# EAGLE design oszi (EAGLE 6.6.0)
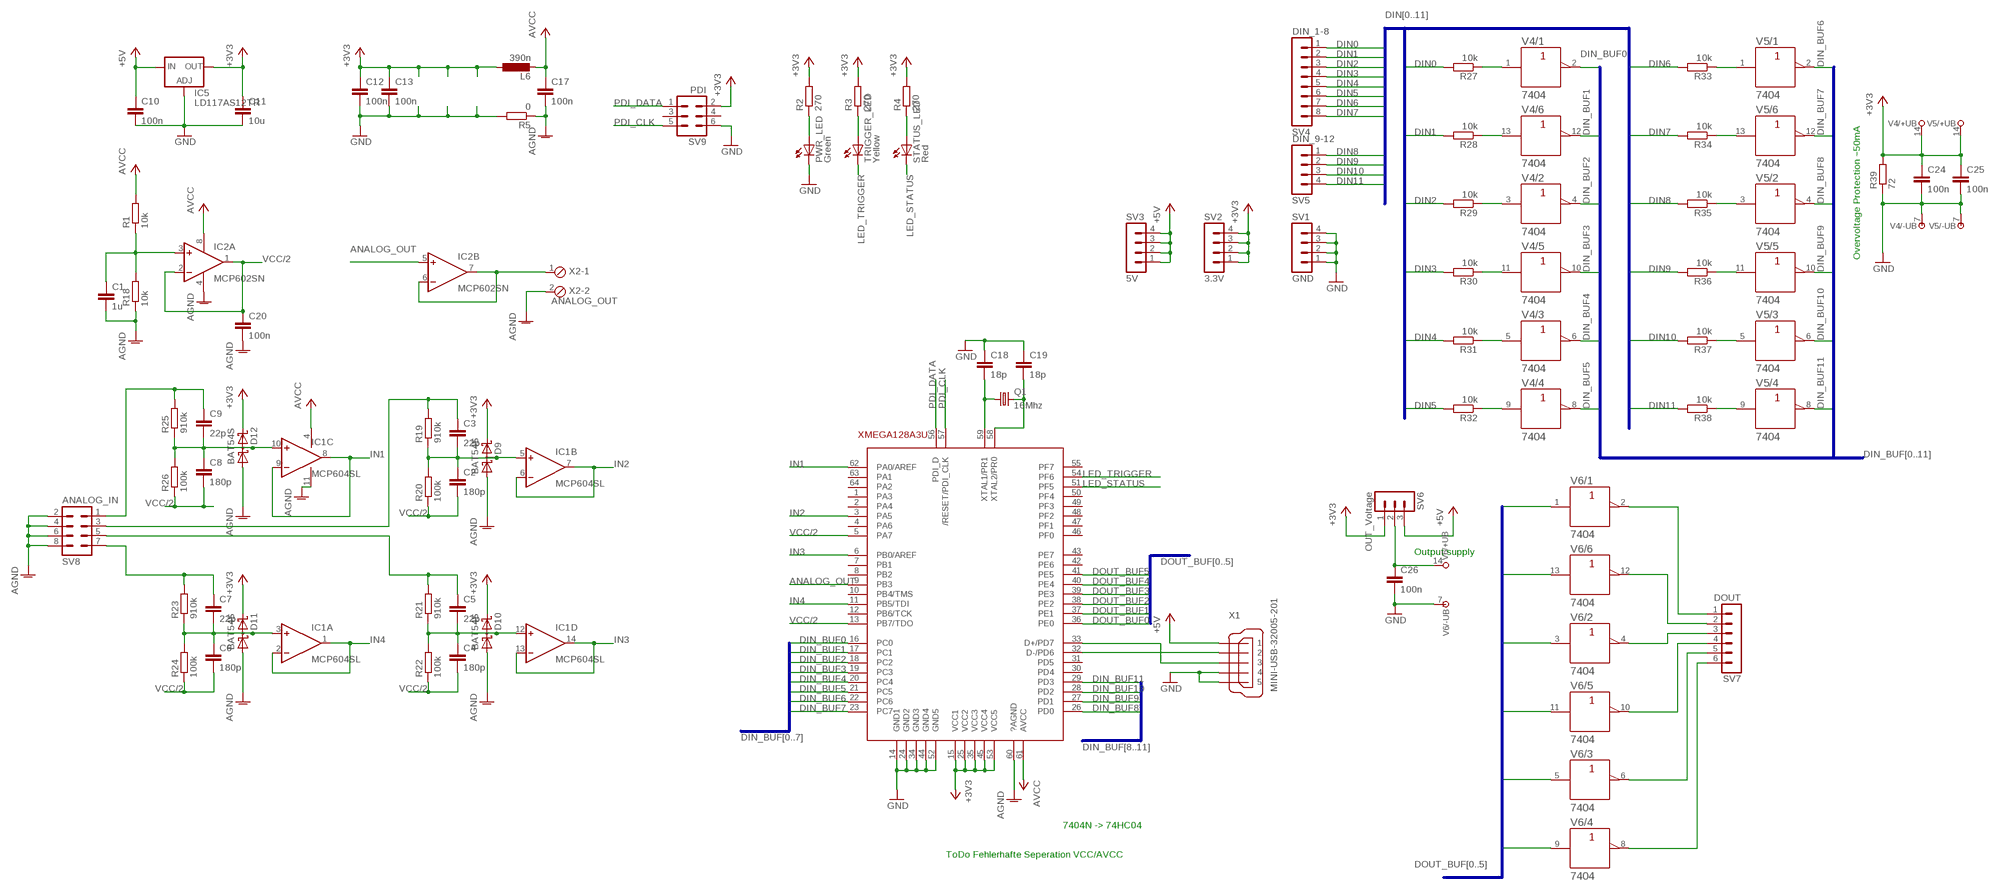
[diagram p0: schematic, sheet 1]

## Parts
C1  1u  C-EUC0805  [C0805]
C2  180p  C-EUC0805  [C0805]
C3  22p  C-EUC0805  [C0805]
C4  180p  C-EUC0805  [C0805]
C5  22p  C-EUC0805  [C0805]
C6  180p  C-EUC0805  [C0805]
C7  22p  C-EUC0805  [C0805]
C8  180p  C-EUC0805  [C0805]
C9  22p  C-EUC0805  [C0805]
C10  100n  C-EUC0805  [C0805]
C11  10u  C-EUC0805  [C0805]
C12  100n  C-EUC0805  [C0805]
C13  100n  C-EUC0805  [C0805]
C17  100n  C-EUC0805  [C0805]
C18  18p  C-EUC0805  [C0805]
C19  18p  C-EUC0805  [C0805]
C20  100n  C-EUC0805  [C0805]
C24  100n  C-EUC0805  [C0805]
C25  100n  C-EUC0805  [C0805]
C26  100n  C-EUC0805  [C0805]
D9  BAT54S  [SOT23]
D10  BAT54S  [SOT23]
D11  BAT54S  [SOT23]
D12  BAT54S  [SOT23]
IC1  MCP604SL  [SO14]
IC2  MCP602SN  [SO08]
IC5  LD117AS12TR  [SOT223]
L6  390n  L-EUL2825P  [L2825P]
PWR_LED  Green  LEDSML0805  [SML0805]
Q1  16Mhz  CRYSTALHC49UP  [HC49UP]
R1  10k  R-EU_R0805  [R0805]
R2  270  R-EU_R0805  [R0805]
R3  270  R-EU_R0805  [R0805]
R4  270  R-EU_R0805  [R0805]
R5  0  R-EU_R0805  [R0805]
R18  10k  R-EU_R0805  [R0805]
R19  910k  R-EU_R0805  [R0805]
R20  100k  R-EU_R0805  [R0805]
R21  910k  R-EU_R0805  [R0805]
R22  100k  R-EU_R0805  [R0805]
R23  910k  R-EU_R0805  [R0805]
R24  100k  R-EU_R0805  [R0805]
R25  910k  R-EU_R0805  [R0805]
R26  100k  R-EU_R0805  [R0805]
R27  10k  R-EU_R0805  [R0805]
R28  10k  R-EU_R0805  [R0805]
R29  10k  R-EU_R0805  [R0805]
R30  10k  R-EU_R0805  [R0805]
R31  10k  R-EU_R0805  [R0805]
R32  10k  R-EU_R0805  [R0805]
R33  10k  R-EU_R0805  [R0805]
R34  10k  R-EU_R0805  [R0805]
R35  10k  R-EU_R0805  [R0805]
R36  10k  R-EU_R0805  [R0805]
R37  10k  R-EU_R0805  [R0805]
R38  10k  R-EU_R0805  [R0805]
R39  72  R-EU_R0805  [R0805]
STATUS_LED  Red  LEDSML0805  [SML0805]
SV1  GND  MA04-1  [MA04-1]
SV2  3.3V  MA04-1  [MA04-1]
SV3  5V  MA04-1  [MA04-1]
SV4  DIN_1-8  MA08-1  [MA08-1]
SV5  DIN_9-12  MA04-1  [MA04-1]
SV6  OUT_Voltage  MA03-1  [MA03-1]
SV7  DOUT  MA06-1  [MA06-1]
SV8  ANALOG_IN  MA04-2  [MA04-2]
SV9  PDI  ML6  [ML6]
TRIGGER_LED  Yellow  LEDSML0805  [SML0805]
U$1  XMEGA128A3U  [TQFP64]
V4  7404  [SO14]
V5  7404  [SO14]
V6  7404  [SO14]
X1  MINI-USB-32005-201  [32005-201]
X2  ANALOG_OUT  MPT2  [2POL254]

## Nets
+3V3: C11.1 C12.1 C13.1 C24.1 C25.1 D9.2(C2) D10.2(C2) D11.2(C2) D12.2(C2) IC5.4(OUT) L6.1 R2.2 R3.2 R4.2 R39.2 SV2.1 SV2.2 SV2.3 SV2.4 SV6.1 SV9.2 U$1.15(VCC1) U$1.25(VCC2) U$1.35(VCC3) U$1.45(VCC4) U$1.53(VCC5) V4.14(/+UB:+UB) V5.14(/+UB:+UB)
+5V: C10.1 IC5.3(IN) SV3.1 SV3.2 SV3.3 SV3.4 SV6.3 X1.1
AGND: C1.2 C17.2 C20.2 D9.1(A1) D10.1(A1) D11.1(A1) D12.1(A1) IC1.11(P:V-) IC2.4(P:V-) R5.1 R18.1 SV8.2 SV8.4 SV8.6 SV8.8 U$1.60(?AGND) X2.2
ANALOG_OUT: IC2.5(B:+IN) U$1.9(PB3)
DIN0: R27.2 SV4.1
DIN1: R28.2 SV4.2
DIN2: R29.2 SV4.3
DIN3: R30.2 SV4.4
DIN4: R31.2 SV4.5
DIN5: R32.2 SV4.6
DIN6: R33.2 SV4.7
DIN7: R34.2 SV4.8
DIN8: R35.2 SV5.1
DIN9: R36.2 SV5.2
DIN10: R37.2 SV5.3
DIN11: R38.2 SV5.4
DIN_BUF0: U$1.16(PC0) V4.2(/1:Y)
DIN_BUF1: U$1.17(PC1) V4.12(/6:Y)
DIN_BUF2: U$1.18(PC2) V4.4(/2:Y)
DIN_BUF3: U$1.19(PC3) V4.10(/5:Y)
DIN_BUF4: U$1.20(PC4) V4.6(/3:Y)
DIN_BUF5: U$1.21(PC5) V4.8(/4:Y)
DIN_BUF6: U$1.22(PC6) V5.2(/1:Y)
DIN_BUF7: U$1.23(PC7) V5.12(/6:Y)
DIN_BUF8: U$1.26(PD0) V5.4(/2:Y)
DIN_BUF9: U$1.27(PD1) V5.10(/5:Y)
DIN_BUF10: U$1.28(PD2) V5.6(/3:Y)
DIN_BUF11: U$1.29(PD3) V5.8(/4:Y)
DOUT_BUF0: U$1.36(PE0) V6.1(/1:A)
DOUT_BUF1: U$1.37(PE1) V6.13(/6:A)
DOUT_BUF2: U$1.38(PE2) V6.3(/2:A)
DOUT_BUF3: U$1.39(PE3) V6.11(/5:A)
DOUT_BUF4: U$1.40(PE4) V6.5(/3:A)
DOUT_BUF5: U$1.41(PE5) V6.9(/4:A)
GND: C10.2 C11.2 C12.2 C13.2 C18.1 C19.1 C24.2 C25.2 C26.2 IC5.1(ADJ) PWR_LED.C R5.2 R39.1 SV1.1 SV1.2 SV1.3 SV1.4 SV9.6 U$1.14(GND1) U$1.24(GND2) U$1.34(GND3) U$1.44(GND4) U$1.52(GND5) V4.7(/-UB:-UB) V5.7(/-UB:-UB) V6.7(/-UB:-UB) X1.4 X1.5
IN1: IC1.8(C:OUT) IC1.9(C:-IN) U$1.62(PA0/AREF)
IN2: IC1.6(B:-IN) IC1.7(B:OUT) U$1.3(PA5)
IN3: IC1.13(D:-IN) IC1.14(D:OUT) U$1.6(PB0/AREF)
IN4: IC1.1(A:OUT) IC1.2(A:-IN) U$1.11(PB5/TDI)
LED_STATUS: STATUS_LED.C U$1.51(PF5)
LED_TRIGGER: TRIGGER_LED.C U$1.54(PF6)
N$1: U$1.32(D-/PD6) X1.2
N$2: U$1.33(D+/PD7) X1.3
N$3: PWR_LED.A R2.1
N$4: C1.1 IC2.3(A:+IN) R1.1 R18.2
N$5: R3.1 TRIGGER_LED.A
N$6: R33.1 V5.1(/1:A)
N$8: R4.1 STATUS_LED.A
N$21: C2.1 C3.2 D9.3(C1A2) IC1.5(B:+IN) R19.1 R20.2
N$24: C4.1 C5.2 D10.3(C1A2) IC1.12(D:+IN) R21.1 R22.2
N$26: C5.1 R21.2 SV8.5
N$27: C6.1 C7.2 D11.3(C1A2) IC1.3(A:+IN) R23.1 R24.2
N$29: C7.1 R23.2 SV8.7
N$30: C8.1 C9.2 D12.3(C1A2) IC1.10(C:+IN) R25.1 R26.2
N$32: C9.1 R25.2 SV8.1
N$33: IC2.6(B:-IN) IC2.7(B:OUT) X2.1
N$34: R27.1 V4.1(/1:A)
N$35: R28.1 V4.13(/6:A)
N$36: R29.1 V4.3(/2:A)
N$37: R30.1 V4.11(/5:A)
N$38: R31.1 V4.5(/3:A)
N$39: R32.1 V4.9(/4:A)
N$41: R34.1 V5.13(/6:A)
N$42: R35.1 V5.3(/2:A)
N$43: R36.1 V5.11(/5:A)
N$44: R37.1 V5.5(/3:A)
N$45: R38.1 V5.9(/4:A)
N$46: C18.2 Q1.1 U$1.59(XTAL1/PR1)
N$47: C26.1 SV6.2 V6.14(/+UB:+UB)
N$48: SV7.1 V6.2(/1:Y)
N$49: SV7.2 V6.12(/6:Y)
N$50: SV7.3 V6.4(/2:Y)
N$51: SV7.4 V6.10(/5:Y)
N$52: SV7.5 V6.6(/3:Y)
N$53: SV7.6 V6.8(/4:Y)
N$54: C3.1 R19.2 SV8.3
N$55: C19.2 Q1.2 U$1.58(XTAL2/PR0)
PDI_CLK: SV9.5 U$1.57(/RESET/PDI_CLK)
PDI_DATA: SV9.1 U$1.56(PDI_D)
VCC: C17.1 IC1.4(P:V+) IC2.8(P:V+) L6.2 R1.2 U$1.61(AVCC) ; supply symbol labelled AVCC
VCC/2: C2.2 C4.2 C6.2 C8.2 C20.1 IC2.1(A:OUT) IC2.2(A:-IN) R20.1 R22.1 R24.1 R26.1 U$1.5(PA7) U$1.13(PB7/TDO)
Unconnected: SV9.3 SV9.4 U$1.1(PA3) U$1.2(PA4) U$1.4(PA6) U$1.7(PB1) U$1.8(PB2) U$1.10(PB4/TMS) U$1.12(PB6/TCK) U$1.30(PD4) U$1.31(PD5) U$1.42(PE6) U$1.43(PE7) U$1.46(PF0) U$1.47(PF1) U$1.48(PF2) U$1.49(PF3) U$1.50(PF4) U$1.55(PF7) U$1.63(PA1) U$1.64(PA2)

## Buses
DIN[0..11]
DIN_BUF[0..11]
DOUT_BUF[0..5]
DIN_BUF[0..7]
DIN_BUF[8..11]

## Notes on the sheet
- Overvoltage Protection ~50mA
- Output supply
- 7404N -> 74HC04
- ToDo Fehlerhafte Seperation VCC/AVCC

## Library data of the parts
C1-C13 C17-C20 C24-C26 = resistor:C-EU: CAPACITOR, European symbol
D9-D12 = diode:BAT54S: Schottky Diodes Pin connection corrected 2011-05-04 Source: Fairchild .. BAT54.pdf
IC1 = linear:MCP604: Quad Op Amp 2.7V to 6.0V Single Supply CMOS Source: http://ww1.microchip.com/downloads/en/DeviceDoc/21314g.pdf
IC2 = linear:MCP602: Single Op Amp 2.7V to 6.0V Single Supply CMOS Source: http://ww1.microchip.com/downloads/en/DeviceDoc/21314g.pdf
IC5 = v-reg:LD117A?*: Low drop fixed and adjustable positive voltage regulators 1 A Source: http://www.st.com/stonline/products/literature/ds/7194/ld1117axx.pdf
L6 = resistor:L-EU: INDUCTOR, European symbol
PWR_LED STATUS_LED TRIGGER_LED = led:LED: LED
Q1 = crystal:CRYSTAL: CRYSTAL; OC_FARNELL: unknown; OC_NEWARK: unknown
R1-R5 R18-R39 = resistor:R-EU_: RESISTOR, European symbol
SV1-SV3 SV5 = con-lstb:MA04-1: PIN HEADER; OC_FARNELL: unknown; OC_NEWARK: unknown
SV4 = con-lstb:MA08-1: PIN HEADER; OC_FARNELL: unknown; OC_NEWARK: unknown
SV6 = con-lstb:MA03-1: PIN HEADER; OC_FARNELL: unknown; OC_NEWARK: unknown
SV7 = con-lstb:MA06-1: PIN HEADER; OC_FARNELL: unknown; OC_NEWARK: unknown
SV8 = con-lstb:MA04-2: PIN HEADER; OC_FARNELL: unknown; OC_NEWARK: unknown
SV9 = con-ml:ML6: HARTING; OC_FARNELL: unknown; OC_NEWARK: unknown
U$1 = Wasle:XMEGA128A3U
V4-V6 = Wasle:74*04: Hex INVERTER
X1 = con-cypressindustries:MINI-USB-: MINI USB-B Conector Source: www.cypressindustries.com; OC_FARNELL: unknown; OC_NEWARK: unknown
X2 = con-phoenix-254:MPT2: PHOENIX CONNECTOR; OC_FARNELL: unknown; OC_NEWARK: unknown

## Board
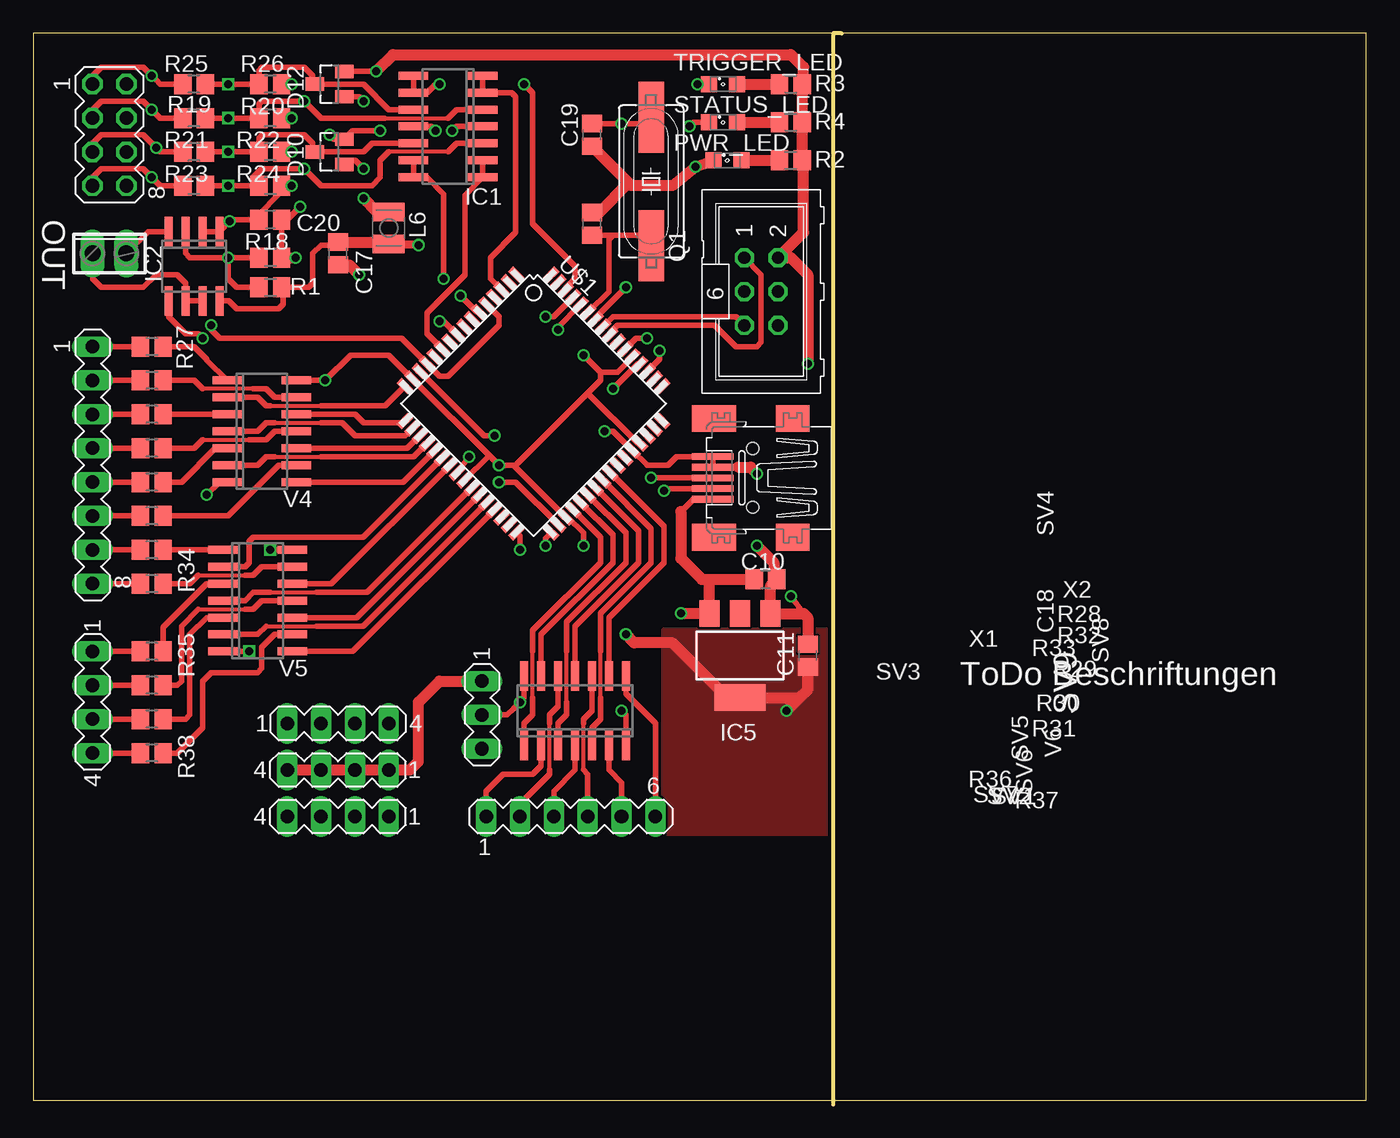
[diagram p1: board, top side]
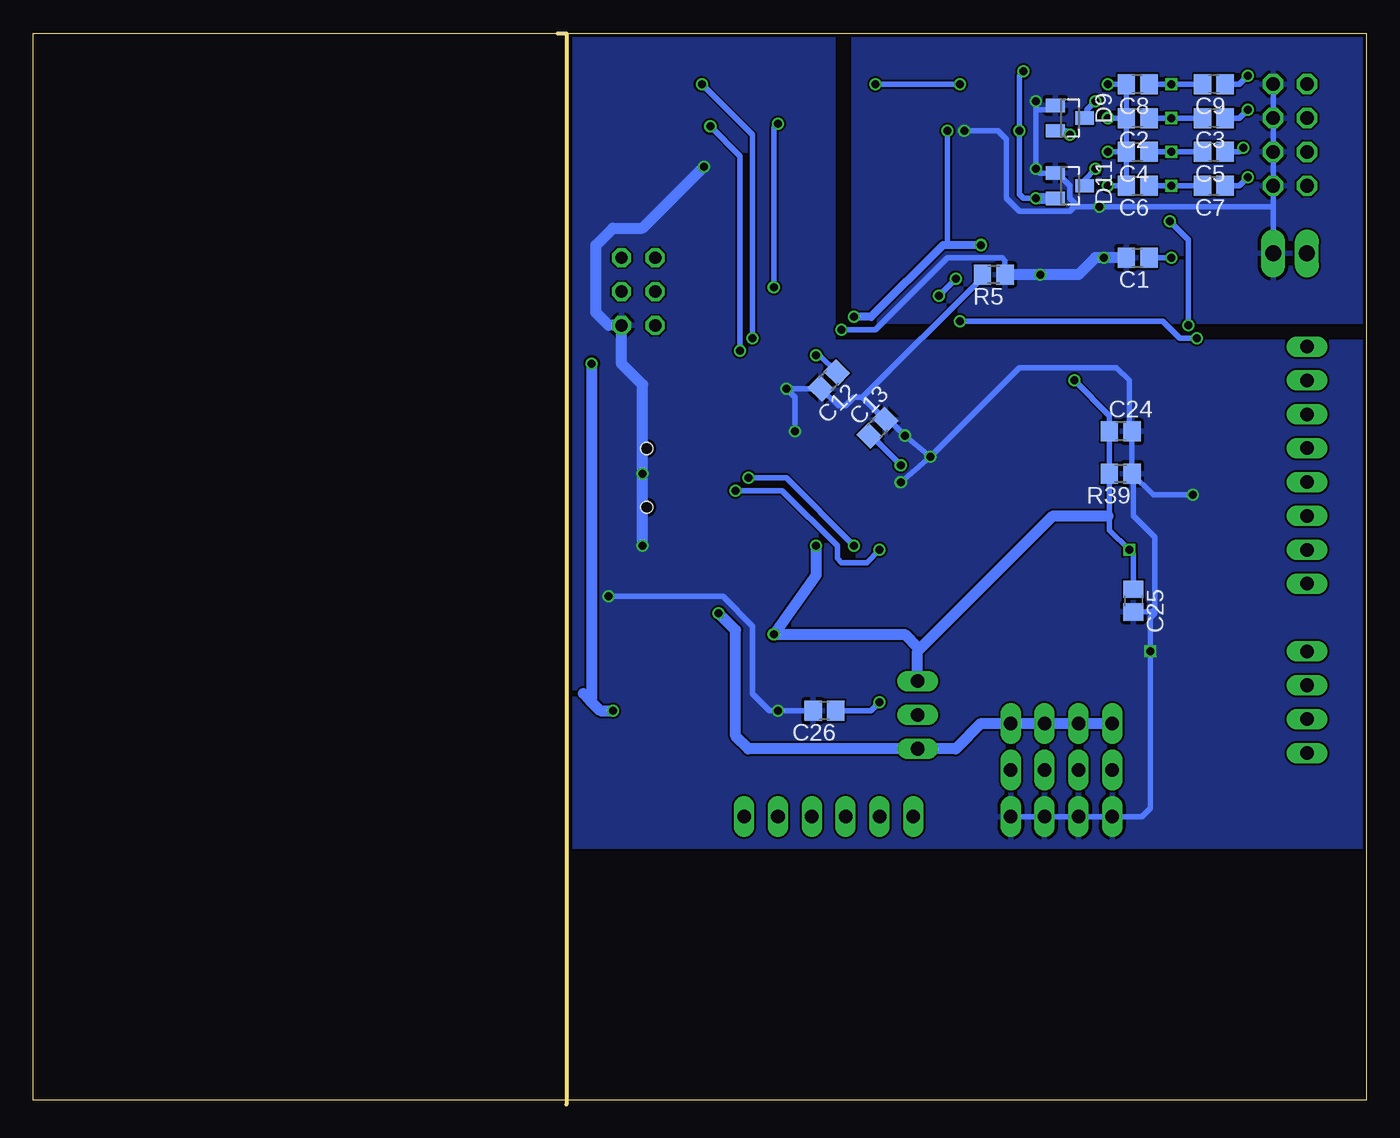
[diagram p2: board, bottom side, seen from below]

Size 100 x 80.33 mm. Coordinates in mm from the lower left corner, seen from the top.
Outline: 60.64,80.33 60.01,80.33 60.01,0
Outline: 0,0.32 100,0.32 100,80.32 0,80.32 0,0.32
Copper layers (1*16): Top 0.035mm / dielectric 1.5mm / Bottom 0.035mm
Design rules "Elecrow_2-layer_eagle_rule": minimum track width 6mil, minimum drill 12mil, track to track 6mil, track to pad 6mil, pad to pad 6mil, via to via 6mil, smd to smd 0mil, copper to edge 10mil, drill to drill 10mil, minimum pad ring 10mil, minimum via ring 6mil, stop-mask expansion 2mil, vias tented up to drill 100mil, thermal gap 10mil

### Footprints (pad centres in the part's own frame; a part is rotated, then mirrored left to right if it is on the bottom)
C0805 = smd 1.3 x 1.5: 1 -0.85,0; 2 0.85,0
SOT23 = smd 1 x 1.4: 1 -0.95,-1.1; 2 0.95,-1.1; 3 0,1.1
SO14 = smd 0.6 x 2.2: 1 -3.81,-2.6; 2 -2.54,-2.6; 3 -1.27,-2.6; 4 0,-2.6; 5 1.27,-2.6; 6 2.54,-2.6; 7 3.81,-2.6; 8 3.81,2.6; 9 2.54,2.6; 10 1.27,2.6; 11 0,2.6; 12 -1.27,2.6; 13 -2.54,2.6; 14 -3.81,2.6
SO08 = smd 0.6 x 2.2: 1 -1.905,-2.6; 2 -0.635,-2.6; 3 0.635,-2.6; 4 1.905,-2.6; 5 1.905,2.6; 6 0.635,2.6; 7 -0.635,2.6; 8 -1.905,2.6
SOT223 = smd 1.5 x 2: 1 -2.3,-3.15; 2 0,-3.15; 3 2.3,-3.15 | smd 3.8 x 2: 4 0,3.15
L2825P = smd 1.4 x 2.4: 1 -1.2,0; 2 1.2,0
SML0805 = smd 1.2 x 1.2: A 1.05,0; C -1.05,0
HC49UP = smd 5.334 x 1.93: 1 -4.826,0; 2 4.826,0
R0805 = smd 1.3 x 1.5: 1 -0.85,0; 2 0.85,0
MA04-1 = drill 1.016 long: 1 -3.81,0; 2 -1.27,0; 3 1.27,0; 4 3.81,0
MA08-1 = drill 1.016 long: 1 -8.89,0; 2 -6.35,0; 3 -3.81,0; 4 -1.27,0; 5 1.27,0; 6 3.81,0; 7 6.35,0; 8 8.89,0
MA03-1 = drill 1.016 long: 1 -2.54,0; 2 0,0; 3 2.54,0
MA06-1 = drill 1.016 long: 1 -6.35,0; 2 -3.81,0; 3 -1.27,0; 4 1.27,0; 5 3.81,0; 6 6.35,0
MA04-2 = drill 1.016 octagon: 1 -3.81,-1.27; 2 -3.81,1.27; 3 -1.27,-1.27; 4 -1.27,1.27; 5 1.27,-1.27; 6 1.27,1.27; 7 3.81,-1.27; 8 3.81,1.27
ML6 = drill 0.914 octagon: 1 -2.54,-1.27; 2 -2.54,1.27; 3 0,-1.27; 4 0,1.27; 5 2.54,-1.27; 6 2.54,1.27
TQFP64 = smd 1.194 x 0.559: 1 -7.76,5.905; 2 -7.76,5.118; 3 -7.76,4.331; 4 -7.76,3.543; 5 -7.76,2.756; 6 -7.76,1.968; 7 -7.76,1.181; 8 -7.76,0.394; 9 -7.76,-0.394; 10 -7.76,-1.181; 11 -7.76,-1.968; 12 -7.76,-2.756; 13 -7.76,-3.543; 14 -7.76,-4.331; 15 -7.76,-5.118; 16 -7.76,-5.905; 33 7.76,-5.905; 34 7.76,-5.118; 35 7.76,-4.331; 36 7.76,-3.543; 37 7.76,-2.756; 38 7.76,-1.968; 39 7.76,-1.181; 40 7.76,-0.394; 41 7.76,0.394; 42 7.76,1.181; 43 7.76,1.968; 44 7.76,2.756; 45 7.76,3.543; 46 7.76,4.331; 47 7.76,5.118; 48 7.76,5.905 | smd 0.559 x 1.194: 17 -5.905,-7.76; 18 -5.118,-7.76; 19 -4.331,-7.76; 20 -3.543,-7.76; 21 -2.756,-7.76; 22 -1.968,-7.76; 23 -1.181,-7.76; 24 -0.394,-7.76; 25 0.394,-7.76; 26 1.181,-7.76; 27 1.968,-7.76; 28 2.756,-7.76; 29 3.543,-7.76; 30 4.331,-7.76; 31 5.118,-7.76; 32 5.905,-7.76; 49 5.905,7.76; 50 5.118,7.76; 51 4.331,7.76; 52 3.543,7.76; 53 2.756,7.76; 54 1.968,7.76; 55 1.181,7.76; 56 0.394,7.76; 57 -0.394,7.76; 58 -1.181,7.76; 59 -1.968,7.76; 60 -2.756,7.76; 61 -3.543,7.76; 62 -4.331,7.76; 63 -5.118,7.76; 64 -5.905,7.76
32005-201 = smd 3.1 x 0.5: 1 3,1.6; 2 3,0.8; 3 3,0; 4 3,-0.8; 5 3,-1.6 | smd 2.5 x 2: M1 -3,-4.45; M2 -3,4.45 | smd 3.3 x 2: M3 2.9,4.45; M4 2.9,-4.45 | hole 0.9: 0,2.2; 0,-2.2
2POL254 = drill 1.2 long: 1 -1.27,0; 2 1.27,0

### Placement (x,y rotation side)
C1  17.14,63.5 180 bottom
C2  17.14,73.98 180 bottom
C3  11.43,73.98 180 bottom
C4  17.14,71.44 180 bottom
C5  11.43,71.44 180 bottom
C6  17.14,68.9 180 bottom
C7  11.43,68.9 180 bottom
C8  17.14,76.52 180 bottom
C9  11.43,76.52 180 bottom
C10  54.93,39.37 0 top
C11  58.1,33.66 90 top
C12  40.31,54.29 225 bottom
C13  36.67,50.74 45 bottom
C17  22.86,63.82 270 top
C18  41.91,66.04 270 top
C19  41.91,72.71 90 top
C20  17.78,66.36 0 top
C24  18.41,50.48 0 bottom
C25  17.46,37.78 270 bottom
C26  40.64,29.53 180 bottom
D9  22.23,73.98 270 bottom
D10  22.23,71.44 90 top
D11  22.23,68.9 270 bottom
D12  22.23,76.52 90 top
IC1  31.11,73.34 90 top
IC2  12.06,62.87 180 top
IC5  53.02,33.66 180 top
L6  26.67,65.72 270 top
PWR_LED  52.07,70.8 0 top
Q1  46.35,69.21 90 top
R1  17.78,61.28 0 top
R2  56.83,70.8 0 top
R3  56.83,76.52 0 top
R4  56.83,73.66 0 top
R5  27.94,62.23 180 bottom
R18  17.78,63.5 180 top
R19  12.06,73.98 180 top
R20  17.78,73.98 180 top
R21  12.06,71.44 180 top
R22  17.78,71.44 180 top
R23  12.06,68.9 180 top
R24  17.78,68.9 180 top
R25  12.06,76.52 180 top
R26  17.78,76.52 180 top
R27  8.89,56.83 180 top
R28  8.89,54.29 180 top
R29  8.89,51.75 180 top
R30  8.89,49.21 180 top
R31  8.89,46.67 180 top
R32  8.89,44.13 180 top
R33  8.89,41.59 180 top
R34  8.89,39.05 180 top
R35  8.89,33.97 180 top
R36  8.89,31.43 180 top
R37  8.89,28.89 180 top
R38  8.89,26.35 180 top
R39  18.41,47.31 180 bottom
STATUS_LED  51.75,73.66 0 top
SV1  22.86,21.59 180 top
SV2  22.86,25.08 180 top
SV3  22.86,28.57 0 top
SV4  4.45,47.94 270 top
SV5  4.45,30.16 270 top
SV6  33.66,29.21 270 top
SV7  40.32,21.59 0 top
SV8  5.71,72.71 270 top
SV9  54.61,60.96 270 top
TRIGGER_LED  51.75,76.52 0 top
U$1  37.54,52.56 315 top
V4  17.14,50.48 270 top
V5  16.83,37.78 270 top
V6  40.64,29.53 0 top
X1  53.98,46.99 180 top
X2  5.71,63.82 0 top

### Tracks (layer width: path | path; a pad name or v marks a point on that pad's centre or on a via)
+3V3  (via drill 0.6)
  Top 0.406: v26.04,73.02 23.96,73.02 D10.2 22.54,72.39 v22.23,72.71 | D12.2 v25.72,77.47 | 34.29,48.58 U$1.15 26.66,56.2 23.81,56.2 v21.91,54.29 V4.14 | 34.29,48.58 34.11,48.58 U$1.25 | 34.29,48.58 v34.92,47.94 36.03,47.94 36.11,47.86 | V5.14 v17.78,41.59 | 36.11,47.86 U$1.35 40.12,44.01 41.27,42.86 v41.27,41.91 | U$1.53 44.97,56.08 43.81,54.93 42.55,54.93 | v41.27,56.2 42.55,54.93 | 42.55,54.93 42.55,54.29 41.59,53.34 | 41.59,53.34 36.11,47.86 | U$1.45 45.35,49.58 41.59,53.34 | R3.2 57.78,76.52
  Top 0.813: SV2.4 SV2.3 SV2.2 SV2.1 28.26,25.08 28.89,25.72 28.89,30.16 30.48,31.75 SV6.1 | 57.49,30.51 IC5.4 53.02,30.48 52.07,30.48 47.94,34.61 45.09,34.61 v44.45,35.24 | 57.49,30.51 58.1,31.11 C11.1 | R3.2 R4.2 R2.2 57.78,71.02 57.78,65.41 SV9.2 56.83,63.5 58.1,62.23 v58.1,55.56 | v25.72,77.47 26.99,78.74 56.83,78.74 57.78,77.79 57.78,76.52 | v56.52,29.53 57.49,30.51 | L6.1 25.79,66.93 v24.77,67.95
  Bottom 0.406: v24.77,67.95 25.72,67.95 26.04,68.26 v26.04,73.02 26.04,77.15 v25.72,77.47 | C25.1 17.46,41.28 v17.78,41.59 19.27,43.08 R39.2 C24.1 19.27,51.65 v21.91,54.29 | v41.27,56.2 41.02,56.2 C12.1 | C13.1 37.13,50.14 v34.92,47.94 | D9.2 22.55,73.03 v22.23,72.71
  Bottom 0.813: 33.66,33.97 33.66,34.29 34.61,35.24 v44.45,35.24 41.27,39.69 v41.27,41.91 | 58.74,30.8 58.26,30.32 | 58.26,30.32 57.47,29.53 v56.52,29.53 | v58.1,55.56 58.1,30.48 58.26,30.32 | v24.77,67.95 D11.2 | SV6.1 33.66,33.97 | 33.66,33.97 23.5,44.13 19.37,44.13
  pour Top (no thermals): 47.31,35.56 59.69,35.56 59.69,20.32 47.31,20.32
+5V  (via drill 0.6)
  Top 0.406: X1.1 49.52,45.39 48.58,44.45
  Top 0.813: 48.58,44.45 48.58,40.96 50.16,39.37 50.8,39.37 | 50.8,39.37 C10.1 | 50.8,39.37 50.72,39.29 IC5.3 50.7,36.83 v48.58,36.83
  Bottom 0.813: v48.58,36.83 47.31,35.56 47.31,27.62 46.35,26.67 SV6.3 30.8,26.67 28.89,28.58 SV3.4 SV3.3 SV3.2 SV3.1
AGND  (via drill 0.6)
  Top 0.406: D12.1 24.45,75.57 v24.77,75.25 | v24.77,70.17 24.13,70.8 23.64,70.8 D10.1 | IC2.4 8.63,65.46 X2.2 | R18.1 C20.2 19.05,66.36 v20,67.31 | v39.37,58.1 39.37,58.3 U$1.60 | IC1.11 29.84,73.34 v30.16,73.02
  Top 0.813: C17.2 23.71,62.97 v24.45,62.23 | R18.1 v19.68,63.5
  Bottom 0.406: SV8.2 SV8.4 SV8.6 SV8.8 6.99,67.31 | v24.77,75.25 24.77,74.61 | 24.77,74.61 23.64,74.61 D9.1 | 24.77,74.61 v24.77,70.17 24.45,69.85 D11.1 23.18,69.85 22.23,68.9 22.23,67.94 21.59,67.31 | 6.99,67.31 X2.2 | 6.99,67.31 v20,67.31 21.59,67.31 | 21.59,67.31 21.91,67.31 22.23,66.99 26.04,66.99 26.99,67.94 26.99,72.39 27.62,73.02 v30.16,73.02 | R5.1 27.09,63.29 27.3,63.5 31.43,63.5 36.83,58.1 v39.37,58.1
  Bottom 0.813: R5.1 v24.45,62.23 21.59,62.23 20.32,63.5 v19.68,63.5 C1.2
  pour Bottom: -0.64,81.6 38.42,81.6 38.42,58.74 -0.64,58.74
ANALOG_OUT  (via drill 0.6)
  Top 0.406: IC2.5 10.16,59.05 11.43,57.79 12.38,57.79 v12.7,57.47 | U$1.9 30.8,58.74 v30.48,58.74
  Bottom 0.406: v12.7,57.47 13.97,57.47 15.24,58.74 v30.48,58.74
DIN0
  Top 0.406: R27.2 SV4.1
DIN1
  Top 0.406: R28.2 SV4.2
DIN2
  Top 0.406: SV4.3 R29.2
DIN3
  Top 0.406: SV4.4 R30.2
DIN4
  Top 0.406: SV4.5 R31.2
DIN5
  Top 0.406: SV4.6 R32.2
DIN6
  Top 0.406: SV4.7 R33.2
DIN7
  Top 0.406: SV4.8 R34.2
DIN8
  Top 0.406: SV5.1 R35.2
DIN9
  Top 0.406: SV5.2 R36.2
DIN10
  Top 0.406: SV5.3 R37.2
DIN11
  Top 0.406: SV5.4 R38.2
DIN_BUF0
  Top 0.305: 17.78,52.39 21.59,52.39
  Top 0.406: V4.2 16.83,53.02 17.46,52.39 17.78,52.39 | 21.59,52.39 26.39,52.39 U$1.16
DIN_BUF1
  Top 0.406: V4.12 24.13,51.75 24.77,51.12 27.74,51.12 U$1.17
DIN_BUF2
  Top 0.305: 18.1,51.12 21.59,51.12
  Top 0.406: V4.4 16.83,50.48 17.46,51.12 18.1,51.12 | 21.59,51.12 23.18,51.12 24.13,50.16 27.9,50.16 U$1.18
DIN_BUF3
  Top 0.406: V4.10 28.06,49.21 U$1.19
DIN_BUF4
  Top 0.305: 18.1,48.58 21.59,48.58
  Top 0.406: V4.6 16.83,47.94 17.46,48.58 18.1,48.58 | 21.59,48.58 28.54,48.58 U$1.20
DIN_BUF5
  Top 0.406: V4.8 27.75,46.67 U$1.21
DIN_BUF6
  Top 0.406: V5.2 15.88,40.32 16.19,40.64 16.19,42.23 16.51,42.54 24.73,42.54 U$1.22
DIN_BUF7
  Top 0.406: V5.12 22.36,39.05 U$1.23
DIN_BUF8
  Top 0.305: 17.78,38.42 21.27,38.42
  Top 0.406: V5.4 15.88,37.78 16.51,38.42 17.78,38.42 | 21.27,38.42 25.06,38.42 U$1.26
DIN_BUF9
  Top 0.406: V5.10 24.27,36.51 U$1.27
DIN_BUF10
  Top 0.305: 17.46,35.88 21.27,35.88
  Top 0.406: V5.6 16.83,35.24 17.46,35.88 | 21.27,35.88 24.75,35.88 U$1.28
DIN_BUF11
  Top 0.406: V5.8 23.96,33.97 U$1.29
DOUT_BUF0
  Top 0.305: 37.47,30.48 37.47,33.97
  Top 0.406: V6.1 36.83,28.58 37.47,29.21 37.47,30.48 | 37.47,33.97 37.47,35.56 42.55,40.64 42.55,42.54 U$1.36
DOUT_BUF1
  Top 0.406: V6.13 38.1,35.24 43.5,40.64 43.5,42.7 U$1.37
DOUT_BUF2
  Top 0.305: 40.01,30.16 40.01,33.97
  Top 0.406: V6.3 39.37,28.58 40.01,29.21 40.01,30.16 | 40.01,33.97 40.01,36.19 44.45,40.64 44.45,42.86 U$1.38
DOUT_BUF3
  Top 0.406: V6.11 40.64,35.88 45.4,40.64 45.4,43.03 U$1.39
DOUT_BUF4
  Top 0.305: 42.55,30.48 42.55,33.97
  Top 0.406: V6.5 41.91,28.26 42.55,28.89 42.55,30.48 | 42.55,33.97 42.55,36.83 46.35,40.64 46.35,43.19 U$1.40
DOUT_BUF5
  Top 0.406: V6.9 43.18,36.51 47.31,40.64 47.31,43.35 U$1.41
GND  (via drill 0.6)
  Top 0.406: U$1.24 31.8,47.35 v32.7,48.58 | v34.61,50.16 33.81,50.16 U$1.14 28.83,54.99 | v16.19,33.97 V5.7 | 52.87,47.79 X1.4 X1.5 48.27,48.59 47.62,47.94 46.04,47.94 46.04,47.96 U$1.44 44.95,49.02 43.5,50.48 v42.86,50.48 | V6.7 44.45,29.21 v44.13,29.53 | U$1.34 36.2,46.67 v34.92,46.67 | U$1.52 45.38,55.54 v43.5,53.66 | v56.83,38.1 57.78,36.83 57.81,36.8 | V4.7 13.97,46.67 v13.02,45.72
  Top 0.813: C11.2 58.1,36.51 57.81,36.8 IC5.1 55.32,38.91 C10.2 55.56,39.58 55.56,40.64 v54.29,41.91 | PWR_LED.C 51.12,70.8 v49.69,70.33 47.94,68.9 44.87,68.9 44.66,69.11 | 44.66,69.11 C19.1 | C18.1 42.44,66.89 44.66,69.11 | 52.87,47.79 53.81,47.79 v54.29,47.31
  Bottom 0.406: R39.1 C24.2 17.78,50.7 17.78,54.29 18.73,55.25 26.04,55.25 v32.7,48.58 | v32.7,48.58 v34.61,50.16 35.79,51.35 C13.2 36.1,51.35 37.78,53.02 | v34.92,46.67 v32.7,48.58 | SV1.1 SV1.2 SV1.3 SV1.4 16.83,21.59 16.19,22.22 v16.19,33.97 16.19,36.51 15.88,36.83 15.98,36.93 16.09,36.93 | C25.2 16.09,36.93 | 16.09,36.93 15.88,37.15 15.88,42.54 17.46,44.13 17.46,47.21 R39.1 | C26.2 v44.13,29.53 44.77,29.53 46.04,30.8 46.04,35.88 48.26,38.1 v56.83,38.1 | 37.78,53.02 38.42,53.02 39.05,52.39 39.61,52.39 C12.2 40.94,53.66 v43.5,53.66 42.86,53.02 v42.86,50.48 | v13.02,45.72 15.98,45.72 R39.1 | R5.2 28.79,62.01 37.78,53.02
  Bottom 0.813: v49.69,70.33 54.29,65.72 56.52,65.72 57.78,64.45 57.78,59.37 56.83,58.42 SV9.6 55.88,55.56 54.29,53.97 v54.29,47.31 v54.29,41.91
  pour Bottom: -0.64,57.15 40.01,57.15 40.01,80.96 60.33,80.96 60.64,80.96 60.64,19.37 -0.64,19.37
IN1  (via drill 0.6)
  Top 0.406: IC1.8 IC1.9 29.53,75.88 30.16,76.52 v30.48,76.52 | U$1.62 39.96,61.23 40.64,61.91 40.64,62.86 37.47,66.04 37.47,75.88 v36.83,76.52
  Bottom 0.406: v36.83,76.52 v30.48,76.52
IN2
  Top 0.406: IC1.7 IC1.6 35.88,75.88 36.2,75.57 36.2,65.41 34.29,63.5 34.29,61.93 U$1.3
IN3  (via drill 0.6)
  Top 0.406: IC1.13 IC1.14 29.53,69.53 30.8,68.26 v30.8,61.91 | U$1.6 33.27,59.44 v32.07,60.64
  Bottom 0.406: v32.07,60.64 v30.8,61.91
IN4
  Top 0.406: IC1.2 IC1.1 32.38,68.2 32.38,62.23 29.53,59.37 29.53,57.79 U$1.11
LED_STATUS  (via drill 0.6)
  Top 0.406: STATUS_LED.C 49.53,73.66 v49.21,73.34 | v46.99,56.51 46.99,55.89 U$1.51
  Bottom 0.406: v49.21,73.34 46.99,71.12 v46.99,56.51
LED_TRIGGER  (via drill 0.6)
  Top 0.406: v49.85,76.52 TRIGGER_LED.C | v46.04,57.47 45.22,57.47 U$1.54
  Bottom 0.406: v46.04,57.47 46.04,72.71 v49.85,76.52
N$1  (via drill 0.6)
  Top 0.406: X1.2 47.46,46.19 v47.31,46.04 | v36.51,41.59 36.51,42.61 U$1.32
  Bottom 0.406: v47.31,46.04 43.81,46.04 39.69,41.91 39.69,40.96 39.37,40.64 37.47,40.64 v36.51,41.59
N$2  (via drill 0.6)
  Top 0.406: X1.3 v46.35,46.99 | v38.42,41.91 38.42,42.47 U$1.33
  Bottom 0.406: v46.35,46.99 43.5,46.99 v38.42,41.91
N$3
  Top 0.813: PWR_LED.A R2.1
N$4  (via drill 0.6)
  Top 0.406: IC2.3 11.43,63.82 11.75,63.5 v14.61,63.5 | v14.61,63.5 R18.2 | R1.1 15.24,61.28 14.61,61.91 v14.61,63.5
  Bottom 0.406: 15.24,63.5 C1.1 v14.61,63.5
N$5
  Top 0.813: TRIGGER_LED.A R3.1
N$6
  Top 0.406: R33.1 V5.1
N$8
  Top 0.813: STATUS_LED.A R4.1
N$21  (via drill 0.6)
  Top 0.305: 26.35,73.98 31.11,73.98
  Top 0.406: R19.1 v14.61,73.98 R20.2 16.93,75.03 17.14,75.25 v20.32,75.25 21.59,73.98 26.35,73.98 | IC1.5 31.75,74.61 31.11,73.98
  Bottom 0.406: C3.2 v14.61,73.98 C2.1 | v20.32,75.25 20.95,74.61 20.95,74.15 D9.3
N$24  (via drill 0.6)
  Top 0.406: R21.1 v14.61,71.44 R22.2 16.93,72.49 17.14,72.71 20.32,72.71 20.95,72.07 20.95,71.61 D10.3 24.77,71.44 25.4,72.07 IC1.12
  Bottom 0.406: C5.2 v14.61,71.44 C4.1
N$26  (via drill 0.6)
  Top 0.406: SV8.5 4.45,72.07 5.08,72.71 8.26,72.71 v9.21,71.76 9.53,71.44 R21.2
  Bottom 0.406: C5.1 9.53,71.44 v9.21,71.76
N$27  (via drill 0.6)
  Top 0.305: 31.11,71.44 26.67,71.44
  Top 0.406: R23.1 v14.61,68.9 R24.2 16.51,69.32 16.51,69.53 17.14,70.17 v20.32,70.17 21.59,68.9 25.4,68.9 26.04,69.53 26.04,70.8 26.67,71.44 | IC1.3 31.75,72.07 31.11,71.44
  Bottom 0.406: C7.2 v14.61,68.9 C6.1 | D11.3 21.12,69.36 v20.32,70.17
N$29  (via drill 0.6)
  Top 0.406: SV8.7 4.45,69.53 5.08,70.17 8.26,70.17 v8.89,69.53 9.53,68.9 R23.2
  Bottom 0.406: C7.1 9.53,68.9 v8.89,69.53
N$30  (via drill 0.6)
  Top 0.406: R25.1 v14.61,76.52 R26.2 16.93,77.57 17.14,77.79 20.32,77.79 20.95,77.15 20.95,76.69 D12.3 24.77,76.52 26.67,74.61 IC1.10
  Bottom 0.406: C9.2 v14.61,76.52 C8.1
N$32  (via drill 0.6)
  Top 0.406: SV8.1 4.45,77.15 5.08,77.79 8.26,77.79 v8.89,77.15 9.21,76.83 9.53,76.52 R25.2
  Bottom 0.406: C9.1 9.53,76.52 v8.89,77.15
N$33
  Top 0.406: IC2.7 IC2.6 11.43,61.6 10.79,62.23 9.21,62.23 8.26,61.28 5.08,61.28 4.45,61.91 X2.1
N$34
  Top 0.406: R27.1 12.06,56.83 13.02,55.88 13.02,55.82 V4.1
N$35
  Top 0.305: 16.51,53.66 12.7,53.66
  Top 0.406: V4.13 18.1,53.02 17.46,53.66 16.51,53.66 | 12.7,53.66 12.06,54.29 R28.1
N$36
  Top 0.406: R29.1 V4.3
N$37
  Top 0.305: 12.7,49.85 16.19,49.85
  Top 0.406: R30.1 12.06,49.21 12.7,49.85 | 16.19,49.85 17.46,49.85 18.1,50.48 V4.11
N$38
  Top 0.406: R31.1 11.11,46.67 13.65,49.21 V4.5
N$39
  Top 0.406: R32.1 14.61,44.13 18.41,47.94 V4.9
N$41
  Top 0.305: 12.38,39.69 15.88,39.69
  Top 0.406: R34.1 11.75,39.05 12.38,39.69 | 15.88,39.69 16.51,39.69 17.14,40.32 V5.13
N$42
  Top 0.406: R35.1 9.74,35.78 13.02,39.05 V5.3
N$43
  Top 0.305: 12.38,37.15 15.88,37.15
  Top 0.406: R36.1 10.79,31.43 11.11,31.75 11.11,35.88 12.38,37.15 | 15.88,37.15 16.51,37.15 17.14,37.78 V5.11
N$44
  Top 0.406: R37.1 11.43,28.89 11.75,29.21 11.75,35.24 13.02,36.51 V5.5
N$45
  Top 0.406: R38.1 10.79,26.35 12.7,28.26 12.7,31.75 13.34,32.39 16.83,32.39 17.14,32.7 17.14,34.29 18.1,35.24 V5.9
N$46
  Top 0.406: C18.2 43.5,65.19 | 43.5,65.19 45.55,65.19 Q1.1 | U$1.59 41.66,59.44 43.18,60.96 43.18,64.87 43.5,65.19
N$47  (via drill 0.6)
  Top 0.406: V6.14 36.83,30.48 v36.51,30.16 36.04,29.69 35.56,29.21 SV6.2
  Bottom 0.406: C26.1 37.15,29.53 v36.51,30.16
N$48
  Top 0.406: SV7.1 33.97,23.49 35.24,24.77 37.47,24.77 38.1,25.4 V6.2
N$49
  Top 0.305: 38.73,25.08 38.73,28.58
  Top 0.406: SV7.2 36.51,22.54 38.73,24.77 38.73,25.08 | 38.73,28.58 38.73,29.21 39.37,29.84 V6.12
N$50
  Top 0.406: SV7.3 39.05,23.49 40.64,25.08 V6.4
N$51
  Top 0.305: 41.27,25.08 41.27,28.58
  Top 0.406: SV7.4 41.59,24.77 41.27,25.08 | 41.27,28.58 41.27,28.89 41.91,29.53 V6.10
N$52
  Top 0.406: SV7.5 44.13,24.13 43.18,25.08 V6.6
N$53
  Top 0.406: SV7.6 46.67,28.58 44.45,30.8 V6.8
N$54  (via drill 0.6)
  Top 0.406: SV8.3 4.45,74.61 5.08,75.25 8.26,75.25 v8.89,74.61 9.53,73.98 R19.2 11.43,73.98
  Bottom 0.406: C3.1 9.53,73.98 v8.89,74.61
N$55  (via drill 0.6)
  Top 0.406: Q1.2 45.87,73.56 v44.13,73.56 C19.2 | U$1.58 42.19,59.01 v44.45,61.28
  Bottom 0.406: v44.45,61.28 44.45,73.24 v44.13,73.56
PDI_CLK
  Top 0.406: U$1.57 42.77,58.33 43.5,59.05 52.7,59.05 SV9.5
PDI_DATA
  Top 0.406: U$1.56 43.3,57.91 43.81,58.42 51.12,58.42 52.7,56.83 54.29,56.83 54.61,57.15 54.61,62.23 SV9.1
VCC  (via drill 0.6)
  Top 0.406: C17.1 22.64,64.45 21.59,64.45 20.95,63.82 20.95,61.6 20.64,61.28 R1.2 18.73,61.18 18.73,60.01 18.41,59.69 15.24,59.69 14.66,60.26 IC2.8 | v38.42,59.05 39.02,59.05 U$1.61 | IC1.4 31.75,73.34 v31.43,73.02
  Top 0.61: L6.2 28.82,64.52 v28.89,64.45
  Top 0.813: C17.1 26.52,64.67 L6.2
  Bottom 0.406: v31.43,73.02 31.43,64.45
  Bottom 0.61: v28.89,64.45 31.43,64.45 31.75,64.45 37.15,59.05 v38.42,59.05
VCC/2  (via drill 0.6)
  Top 0.406: 18.41,68.68 18.41,68.26 16.93,66.78 C20.1 14.86,66.36 v14.73,66.23 IC2.1 IC2.2 | 18.41,68.68 R24.1 | U$1.5 34.92,59.07 34.92,58.42 31.11,54.61 30.48,54.61 U$1.13 27.62,57.47 13.97,57.47 13.34,58.1 v13.34,58.42 | R26.1 v19.37,76.52 | R20.1 v19.37,73.98 | R22.1 v19.37,71.44 | 18.41,68.68 19.15,68.68 v19.37,68.9
  Bottom 0.406: C2.2 C8.2 v19.37,76.52 | C2.2 C4.2 | C4.2 C6.2 v19.37,68.9 | v13.34,58.42 13.34,64.83 v14.73,66.23 | v19.37,73.98 C2.2 | v19.37,71.44 C4.2

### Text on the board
tNames: OUT | ToDo Beschriftungen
